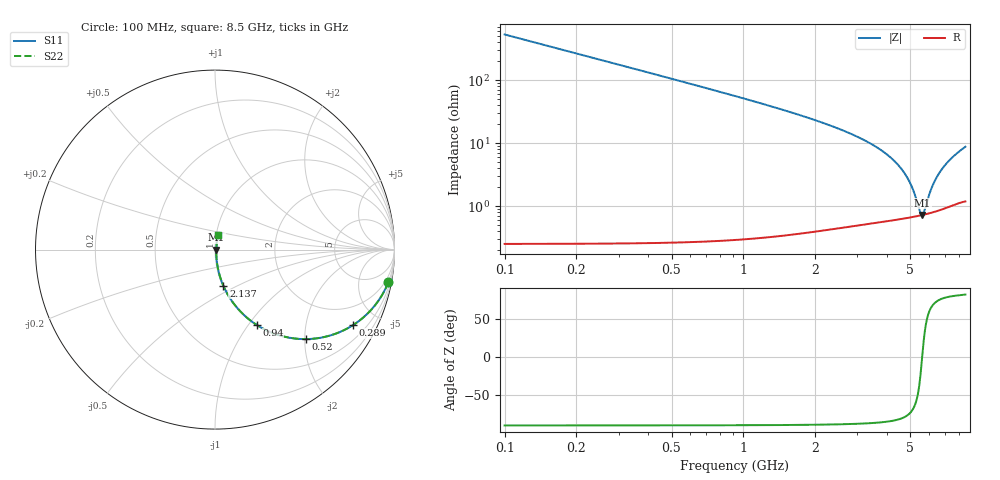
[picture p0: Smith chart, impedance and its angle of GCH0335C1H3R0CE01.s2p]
!Murata Part Number: GCH0335C1H3R0CE01
!These Parameters are Measured in Series Mode Connection
!Data Generated on Mar 13, 2026
!  o--ll--o
!Port1  Port2
!  o------o
!Operation Temp=25[degC], DC Bias Voltage=0[V]
!Freq. Start=100[MHz] Stop=9[GHz] 401[Steps]
# Hz S RI R 50
!Freq.(Hz) S11(Real) S11(Imag) S21(Real) S21(Imag) S12(Real) S12(Imag) S22(Real) S22(Imag)
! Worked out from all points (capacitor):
!   401 points, 100 MHz to 8.5 GHz, reference 50 ohm
!   read as one part in series: C = 3 pF near 142 MHz
!   lowest |Z| = 721 mohm at 5.602 GHz (marker M1)
!   series resonance near 5.603 GHz, so ESL is about 270 pH
!   S11 on the Smith chart (normalised r, x): 100 MHz: 1, -11; 289 MHz: 1.01, -3.66; 520 MHz: 1.01, -2.02; 940 MHz: 1.01, -1.10; 2.137 GHz: 1.01, -0.42; 8.5 GHz: 1.02, +0.17
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1e8  0.9656 -0.1821  0.0344 0.1821  0.0344 0.1821  0.9656 -0.1821
2.05e8  0.8695 -0.3363  0.1305 0.3363  0.1305 0.3363  0.8695 -0.3363
2.89e8  0.7699 -0.4202  0.2301 0.4202  0.2301 0.4202  0.7699 -0.4202
3.94e8  0.6419 -0.4785  0.3581 0.4785  0.3581 0.4785  0.6419 -0.4785
5.2e8  0.5055 -0.4987  0.4945 0.4987  0.4945 0.4987  0.5055 -0.4987
7.09e8  0.3518 -0.4757  0.6482 0.4757  0.6482 0.4757  0.3518 -0.4757
9.4e8  0.2322 -0.4196  0.7678 0.4196  0.7678 0.4196  0.2322 -0.4196
1.507e9  0.0986 -0.2929  0.9014 0.2929  0.9014 0.2929  0.0986 -0.2929
2.137e9  0.0465 -0.2011  0.9535 0.2011  0.9535 0.2011  0.0465 -0.2011
2.914e9  0.0219 -0.1292  0.9781 0.1292  0.9781 0.1292  0.0219 -0.1292
4.3e9  0.00852 -0.0503  0.9915 0.0503  0.9915 0.0503  0.00852 -0.0503
4.657e9  0.0075 -0.0351  0.9925 0.0351  0.9925 0.0351  0.0075 -0.0351
4.951e9  0.00708 -0.0234  0.9929 0.0234  0.9929 0.0234  0.00708 -0.0234
5.182e9  0.00696 -0.0148  0.993 0.0148  0.993 0.0148  0.00696 -0.0148
5.497e9  0.00706 -0.00362  0.9929 0.00362  0.9929 0.00362  0.00706 -0.00362
5.602e9  0.00716 -2.58e-05  0.9928 2.58e-05  0.9928 2.58e-05  0.00716 -2.58e-05
5.707e9  0.00729 0.00351  0.9927 -0.00351  0.9927 -0.00351  0.00729 0.00351
6.022e9  0.00784 0.0138  0.9922 -0.0138  0.9922 -0.0138  0.00784 0.0138
6.295e9  0.00852 0.0224  0.9915 -0.0224  0.9915 -0.0224  0.00852 0.0224
6.652e9  0.00967 0.0332  0.9903 -0.0332  0.9903 -0.0332  0.00967 0.0332
7.114e9  0.0116 0.0465  0.9884 -0.0465  0.9884 -0.0465  0.0116 0.0465
8.5e9  0.0189 0.0841  0.9811 -0.0841  0.9811 -0.0841  0.0189 0.0841
